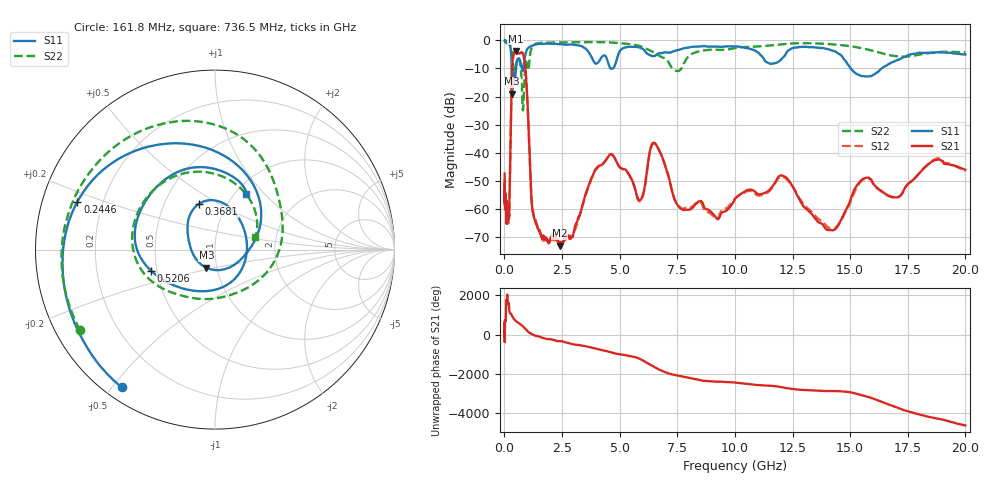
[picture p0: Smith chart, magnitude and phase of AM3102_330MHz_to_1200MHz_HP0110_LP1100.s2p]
! Date/Time: Tue, Sep 11, 2018 5:15 PM
! Network Analyzer: Agilent Technologies E8362B Rev: A.07.50.63
! Sweep from 0.010 to 20.000 GHz, 1601 Points, Sweep Type: LOG
! Power Supply: 4.949 V, 0.001 A
# Hz S DB R 50
!freq MagS11 AngS11 MagS21 AngS21 MagS12 AngS12 MagS22 AngS22
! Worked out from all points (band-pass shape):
!   1601 points, 10 MHz to 20 GHz, reference 50 ohm
!   highest |S21| = -3.73 dB at 484.8 MHz (marker M1); lowest = -73.1 dB at 2.404 GHz (marker M2)
!   |S21| within 3 dB of the highest: 362.1 MHz to 863.6 MHz (501.5 MHz wide, 81.8 % of centre)
!   lowest |S11| = -19.0 dB at 337.9 MHz (marker M3), VSWR 1.25, Z = 44.5 - j9.12 ohm
!   |S11| at or under -10 dB: 314.8 MHz to 503.8 MHz (189 MHz wide, 46.2 % of centre); 4.612 GHz to 4.697 GHz (85.33 MHz wide, 1.83 % of centre); 15.03 GHz to 16.37 GHz (1.343 GHz wide, 8.56 % of centre)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
!   |S22| runs from -24.9 to -0.3 dB; largest |S21 - S12| = 0.011
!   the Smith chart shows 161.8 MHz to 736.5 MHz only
!   S11 on the Smith chart (normalised r, x): 161.8 MHz: 0.05, -0.53; 244.6 MHz: 0.11, +0.17; 368.1 MHz: 0.74, +0.41; 520.6 MHz: 0.46, -0.13; 736.5 MHz: 1.13, +0.79
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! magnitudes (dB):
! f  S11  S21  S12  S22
! 10 MHz  0.0  -47.4  -52.7  -0.3
! 35.55 MHz  0.0  -58.2  -57.7  -0.5
! 126.4 MHz  -0.4  -63.3  -62.1  -1.0
! 161.8 MHz  -0.7  -61.1  -64.0  -1.2
! 244.6 MHz  -1.8  -48.0  -47.9  -1.7
! 337.9 MHz  -19.0  -9.5  -9.5  -6.1
! 368.1 MHz  -11.4  -6.3  -6.4  -8.4
! 447.2 MHz  -14.2  -3.9  -3.9  -11.1
! 484.8 MHz  -11.8  -3.7  -3.8  -9.8
! 520.6 MHz  -8.5  -4.0  -4.1  -7.9
! 736.5 MHz  -9.0  -4.3  -4.3  -12.6
! 942.8 MHz  -4.1  -13.4  -13.5  -7.6
! 1.219 GHz  -1.9  -60.2  -60.6  -2.1
! 1.59 GHz  -1.3  -69.4  -69.2  -0.9
! 2.404 GHz  -1.4  -73.1  -72.6  -0.7
! 4.543 GHz  -9.0  -40.9  -40.8  -0.7
! 5.652 GHz  -2.3  -52.3  -52.6  -1.6
! 6.549 GHz  -5.4  -36.8  -36.9  -4.6
! 7.734 GHz  -2.9  -60.3  -60.0  -9.3
! 12.09 GHz  -6.1  -48.2  -48.6  -1.3
! 14.07 GHz  -3.2  -67.5  -66.7  -1.3
! 20 GHz  -5.0  -46.1  -46.6  -4.2
